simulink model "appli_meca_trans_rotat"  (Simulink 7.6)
settings: Solver=ode15s  StartTime=0.0  StopTime=2  MaxStep=0.2  RelTol=1e-3
StopFcn:
  | close all, clc
  | load couple_pos_vit_rotat.mat
  | load couple_pos_vit_trans.mat
  | subplot 211
  | plot(x(1,:),x(4,:))
  | axis([0 2 -0.2 1.2])
  | title('Système rotationnel')
  | gtext('Couple appliqué')
  | grid
  | subplot 212
  | plot(x(1,:), x(2,:),x(1,:),x(3,:))
  | grid
  | gtext('Position angulaire')
  | gtext('Vitesse angulaire')
  | 
  | figure
  | plot(y(1,:), y(3,:),y(1,:),y(4,:))
  | title('Système linéaire')
  | grid
  | gtext('Position linéaire')
  | gtext('Vitesse linéaire')
undefined symbols (not defined in the file or in its folder): sigbuilder_block
libraries: fl_lib x11, nesl_utility x7

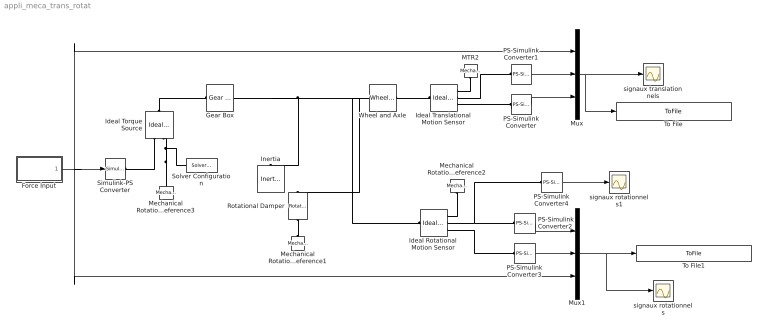
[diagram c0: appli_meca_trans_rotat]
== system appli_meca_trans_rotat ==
  Force Input : Subsystem  Tag=STV Subsys  LoadFcn=sigbuilder_block('load');  StartFcn=sigbuilder_block('start');  StopFcn=sigbuilder_block('stop');  ClipboardFcn=sigbuilder_block('clipboard');
  Gear Box : fl_lib/Mechanical/Mechanisms/Gear Box  Tag=Factory Generic  DialogController=NetworkEngine.DynNeDlgSource  SystemSampleTime=-1  ratio=5  t_in_Log=off  t_out_Log=off  LocalVarNames=|torque_inp|ang_velocity_inp|power  LocalVarDescs=|Input shaft torque (N*m)|Input shaft angular velocity (rad/s)|Power transmitted by the box (W)  LocalVarLogging=[0 0 0]
  Ideal Rotational Motion Sensor : fl_lib/Mechanical/Mechanical Sensors/Ideal Rotational Motion Sensor  DialogController=NetworkEngine.DynNeDlgSource  SystemSampleTime=-1  offset=0 rad  w_Log=off  t_Log=off  phi_Log=off  LocalVarNames=|w|t|phi  LocalVarDescs=|w|t|phi  LocalVarLogging=[0 0 0]
  Ideal Torque Source : fl_lib/Mechanical/Mechanical Sources/Ideal Torque Source  DialogController=NetworkEngine.DynNeDlgSource  SystemSampleTime=-1  w_Log=off  t_Log=off  LocalVarNames=|w|t  LocalVarDescs=|w|t  LocalVarLogging=[0 0]
  Ideal Translational Motion Sensor : fl_lib/Mechanical/Mechanical Sensors/Ideal Translational Motion Sensor  Tag=Factory Generic  DialogController=NetworkEngine.DynNeDlgSource  SystemSampleTime=-1  offset=0 m  v_Log=off  f_Log=off  x_Log=off  LocalVarNames=|v|f|x  LocalVarDescs=|v|f|x  LocalVarLogging=[]
  Inertia : fl_lib/Mechanical/Rotational Elements/Inertia  DialogController=NetworkEngine.DynNeDlgSource  SystemSampleTime=-1  inertia=0.001 kg*m^2  initial_velocity=0 rad/s  t_Log=off  LocalVarNames=|t  LocalVarDescs=|t  LocalVarLogging=0
  MTR2 : fl_lib/Mechanical/Translational Elements/Mechanical Translational Reference  Tag=Factory Generic  DialogController=NetworkEngine.DynNeDlgSource  SystemSampleTime=-1  f_Log=off  LocalVarNames=|f  LocalVarDescs=|f  LocalVarLogging=[]
  Mechanical Rotational Reference1 : fl_lib/Mechanical/Rotational Elements/Mechanical Rotational Reference  DialogController=NetworkEngine.DynNeDlgSource  SystemSampleTime=-1  t_Log=off  LocalVarNames=|t  LocalVarDescs=|t  LocalVarLogging=0
  Mechanical Rotational Reference2 : fl_lib/Mechanical/Rotational Elements/Mechanical Rotational Reference  DialogController=NetworkEngine.DynNeDlgSource  SystemSampleTime=-1  t_Log=off  LocalVarNames=|t  LocalVarDescs=|t  LocalVarLogging=0
  Mechanical Rotational Reference3 : fl_lib/Mechanical/Rotational Elements/Mechanical Rotational Reference  DialogController=NetworkEngine.DynNeDlgSource  SystemSampleTime=-1  t_Log=off  LocalVarNames=|t  LocalVarDescs=|t  LocalVarLogging=0
  Mux : Mux  Inputs=3
  Mux1 : Mux  Inputs=3
  PS-Simulink Converter{,1..4} (5 alike) : nesl_utility/PS-Simulink Converter  DialogController=NetworkEngine.DynNeUtilDlgSource  SystemSampleTime=-1  PhysicalDomain=network_engine_domain  LeftPortType=input  RightPortType=output  SubClassName=ps_output  Unit=1  AffineConversion=off
  Rotational Damper : fl_lib/Mechanical/Rotational Elements/Rotational Damper  DialogController=NetworkEngine.DynNeDlgSource  SystemSampleTime=-1  D=0.01 N*m/(rad/s)  t_Log=off  w_Log=off  LocalVarNames=|t|w  LocalVarDescs=|t|w  LocalVarLogging=[0 0]
  Simulink-PS Converter : nesl_utility/Simulink-PS Converter  DialogController=NetworkEngine.DynNeUtilDlgSource  SystemSampleTime=-1  PhysicalDomain=network_engine_domain  LeftPortType=input  RightPortType=output  SubClassName=ps_input  Unit=1  AffineConversion=off  InputFilterTimeConstant=.001  UdotUserProvided=0
  Solver Configuration : nesl_utility/Solver Configuration  DialogController=NetworkEngine.DynNeUtilDlgSource  SystemSampleTime=-1  PhysicalDomain=network_engine_domain  LeftPortType=input  RightPortType=generic  SubClassName=solver  Accelerate=off  Profile=off  ResidualTolerance=1e-9  MaxNonlinIter=12  MaxModeIter=2  DoFixedCost=off  UseLocalSampling=off  DoDC=off  LinearAlgebra=Full  LocalSolverSampleTime=.001  LocalSolverChoice=NE_BACKWARD_EULER_ADVANCER  UseLocalSolver=off
  To File : ToFile  Filename=couple_pos_vit_trans  MatrixName=y
  To File1 : ToFile  Filename=couple_pos_vit_rotat  MatrixName=x
  Wheel and Axle : fl_lib/Mechanical/Mechanisms/Wheel and Axle  Tag=Factory Generic  DialogController=NetworkEngine.DynNeDlgSource  SystemSampleTime=-1  R=0.5 m  or=1  torque_A_Log=off  force_P_Log=off  ang_velocity_Log=off  velocity_Log=off  LocalVarNames=|torque_A|force_P|ang_velocity|velocity  LocalVarDescs=|Axle torque (N*m)|Periphery force (N)|Axle angular velocity (rad/s)|Periphery velocity (m/s)  LocalVarLogging=[0 0 0 0]
  signaux rotationnels : Scope
  signaux rotationnels1 : Scope
  signaux translationnels : Scope
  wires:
  Force Input/1(Signal 2) -> Simulink-PS Converter/1, Mux/1, Mux1/3
  PS-Simulink Converter/1 -> Mux/3
  PS-Simulink Converter1/1 -> Mux/2
  Mux/1 -> signaux translationnels/1, To File/1
  PS-Simulink Converter2/1 -> Mux1/1
  PS-Simulink Converter3/1 -> Mux1/2
  Mux1/1 -> To File1/1, signaux rotationnels/1
  PS-Simulink Converter4/1 -> signaux rotationnels1/1
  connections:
  Ideal Rotational Motion Sensor/LConn1 -- Wheel and Axle/LConn1 -- Gear Box/RConn1 -- Inertia/LConn1 -- Rotational Damper/LConn1
  Ideal Translational Motion Sensor/LConn1 -- Wheel and Axle/RConn1
  PS-Simulink Converter/LConn1 -- Ideal Translational Motion Sensor/RConn3
  MTR2/LConn1 -- Ideal Translational Motion Sensor/RConn1
  Ideal Translational Motion Sensor/RConn2 -- PS-Simulink Converter1/LConn1
  Mechanical Rotational Reference1/LConn1 -- Rotational Damper/RConn1
  Ideal Rotational Motion Sensor/RConn2 -- PS-Simulink Converter2/LConn1 -- PS-Simulink Converter4/LConn1
  Mechanical Rotational Reference2/LConn1 -- Ideal Rotational Motion Sensor/RConn1
  Ideal Rotational Motion Sensor/RConn3 -- PS-Simulink Converter3/LConn1
  Ideal Torque Source/RConn1 -- Simulink-PS Converter/RConn1
  Ideal Torque Source/RConn2 -- Mechanical Rotational Reference3/LConn1 -- Solver Configuration/RConn1
  Ideal Torque Source/LConn1 -- Gear Box/LConn1

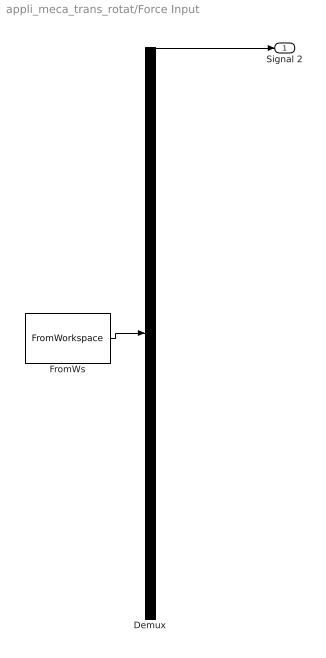
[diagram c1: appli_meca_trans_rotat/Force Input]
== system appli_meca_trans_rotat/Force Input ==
  Demux : Demux  Tag=STV Demux  Outputs=1
  FromWs : FromWorkspace  Tag=STV FromWs  VariableName=tuvar  SampleTime=0  SigBuilderData=DataTag0  VnvData=DataTag1
  Signal 2 : Outport  Tag=STV Outport
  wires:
  FromWs/1 -> Demux/1
  Demux/1 -> Signal 2/1
